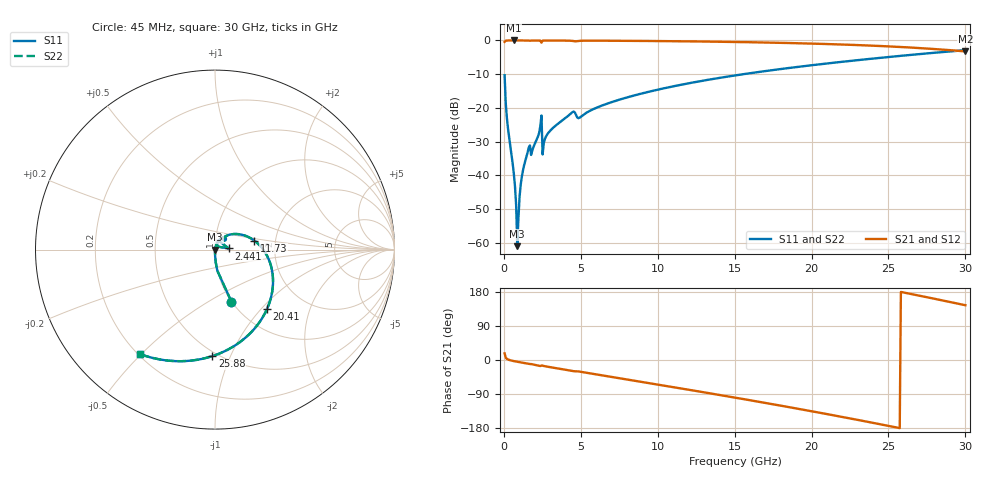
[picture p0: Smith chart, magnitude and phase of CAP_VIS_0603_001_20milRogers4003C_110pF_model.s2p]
! S-parameter model data by Modelithics Inc.  support@modelithics.com  813-866-6335  Tampa FL USA
! S-Parameter data specifications:
! Substrate: 20-mil Rogers 4003C, substrate thickness, H=0.508mm, Dielectric constant, Er=3.75
! PCB Mounting Pad Footprint: Pad width, PadW=0.90mm , Pad length, PadL=1.00mm , Pad gap, PadG (edge-to-edge)=1.00mm , Reference planes=3.0mm apart
! Created Wed Nov 18 13:31:34 2015
# hz S ma R 50
! 2 Port Network Data from SP1.SP block
! freq  magS11  angS11  magS21  angS21  magS12  angS12  magS22  angS22
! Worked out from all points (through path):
!   401 points, 45 MHz to 30 GHz, reference 50 ohm
!   highest |S21| = -0.01 dB at 644.1 MHz (marker M1); lowest = -3.3 dB at 30 GHz (marker M2)
!   group delay of S21, straight-line fit = 19.9 ps
!   lowest |S11| = -61.0 dB at 868.8 MHz (marker M3), VSWR 1.00, Z = 50.1 - j0.0616 ohm
!   |S11| at or under -10 dB: start of sweep to 15.58 GHz
!   |S22| runs from -61.0 to -2.9 dB; largest |S21 - S12| = 0
!   S11 on the Smith chart (normalised r, x): 45 MHz: 1.00, -0.64; 2.441 GHz: 1.17, +0.01; 11.73 GHz: 1.55, +0.16; 20.41 GHz: 1.32, -1.08; 25.88 GHz: 0.47, -0.86; 30 GHz: 0.21, -0.49
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4.5e7  0.3045 -72.5  0.9523 17.5  0.9523 17.5  0.3045 -72.5
2.696625e8  0.04851 -88.2  0.9984 1.3  0.9984 1.3  0.04851 -88.2
6.441e8  0.0106 -89.7  0.9993 -2.9  0.9993 -2.9  0.0106 -89.7
7.189875e8  0.006878 -88.3  0.9993 -3.5  0.9993 -3.5  0.006878 -88.3
8.687625e8  0.0008881 -43.9  0.9992 -4.7  0.9992 -4.7  0.0008881 -43.9
1.018538e9  0.004833 75.3  0.9992 -5.8  0.9992 -5.8  0.004833 75.3
1.2432e9  0.01193 78.4  0.999 -7.4  0.999 -7.4  0.01193 78.4
1.54275e9  0.02198 76.1  0.998 -9.6  0.998 -9.6  0.02198 76.1
1.917188e9  0.02619 74.2  0.9977 -11.9  0.9977 -11.9  0.02619 74.2
2.291625e9  0.04271 71.8  0.9964 -14.9  0.9964 -14.9  0.04271 71.8
2.4414e9  0.07702 4.6  0.9268 -14.7  0.9268 -14.7  0.07702 4.6
2.666062e9  0.03461 70.6  0.9974 -16.4  0.9974 -16.4  0.03461 70.6
4.388475e9  0.08405 55.6  0.9875 -28.6  0.9875 -28.6  0.08405 55.6
5.062462e9  0.07577 52.9  0.9896 -31.7  0.9896 -31.7  0.07577 52.9
1.007992e10  0.1878 23.9  0.9789 -65.4  0.9789 -65.4  0.1878 23.9
1.172745e10  0.2249 12.8  0.9708 -76.5  0.9708 -76.5  0.2249 12.8
1.50225e10  0.3026 -9.8  0.9488 -99.3  0.9488 -99.3  0.3026 -9.8
2.003996e10  0.4297 -45.9  0.8974 -135.5  0.8974 -135.5  0.4297 -45.9
2.04144e10  0.4396 -48.7  0.8925 -138.3  0.8925 -138.3  0.4396 -48.7
2.505742e10  0.5693 -84.7  0.815 -174.3  0.815 -174.3  0.5693 -84.7
2.588119e10  0.5935 -91.4  0.7973 179.0  0.7973 179.0  0.5935 -91.4
3e10  0.7172 -125.9  0.6874 144.5  0.6874 144.5  0.7172 -125.9
